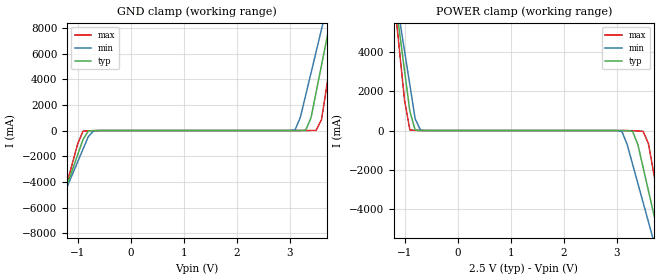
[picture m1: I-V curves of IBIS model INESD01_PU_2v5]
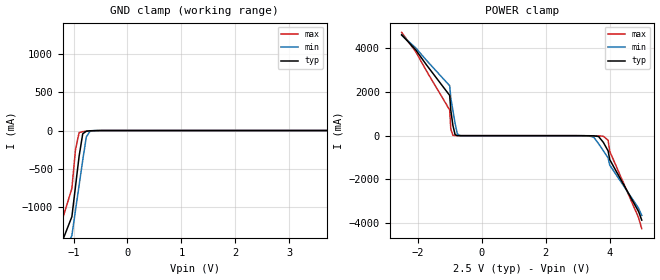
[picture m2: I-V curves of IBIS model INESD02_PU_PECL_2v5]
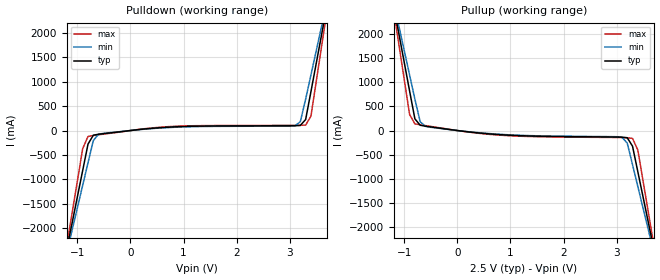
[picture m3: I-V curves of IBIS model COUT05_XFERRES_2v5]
|   This file is an IBIS representation of the   |
|   Integrated Devices Technology, Inc.   |
|   ICS83947I-147   |
|   Low Skew, 1-to-9 LVCMOS/LVTTL Fanout Buffer   |
[IBIS Ver]   4.1
[File name]   83947i_147.ibs
[File Rev]   1.0
[Date]   12 Jun 2009 | Last modified
|   July 26 2002 | Generated
[Source]   Originated at Integrated Devices Technology, Inc.
[Disclaimer]
IDT hereby grants the user of this IBIS model a non-exclusive,
nontransferable license to use this IBIS model under the following terms.
Before using this IBIS model, the user should read this license.
If the user does not accept these terms,  the IBIS model should be
returned to IDT within 30 days.
   The user is granted this license only to use the IBIS model and
is not granted rights to sell, load, rent, lease or license the IBIS
model in whole or in part, or in modified form to anyone other than
user. User may modify the IBIS model to suit its specific
applications but rights to derivative works and such modifications
shall belong to IDT.
   This IBIS model is provided on an "AS IS" basis and IDT makes
absolutely no warranty with respect to the information contained
herein. IDT DISCLAIMS AND CUSTOMER WAIVES ALL WARRANTIES, EXPRESS
OR IMPLIED, INCLUDING WARRANTIES OF MERCHANTABILITY OR FITNESS FOR
A PARTICULAR PURPOSE. The entire risk as to quality and performance
is with the Customer. ACCORDINGLY, IN NO EVENT SHALL THE COMPANY BE
LIABLE FOR ANY DAMAGES, WHETHER IN CONTRACT OR TORT,INCLUDING ANY
LOST PROFITS OR OTHER INCIDENTAL, CONSEQUENTIAL, EXEMPLARY, OR
PUNITIVE DAMAGES ARISING OUT OF THE USE OR APPLICATION OF THE IBIS
model provided in this package. Further, IDT reserves the right to
make changes without notice to any product herein to improve
reliability, function, or design. IDT does not convey any license
under patent rights or any other intellectual property rights,
including those of third parties.
   IDT is not obligated to provide maintenance or support
for the licensed IBIS model.
[Copyright]   Copyright 2002 by Integrated Devices Technology, Inc.
[Component]   ICS83947I-147
[Manufacturer] Integrated Devices Technology, Inc.
[Package]
|LQFP32
|lead + wire   typ   min   max
R_pkg   220.4m   212.5m   238m
L_pkg   1.841n   1.708n   1.974n
C_pkg   0.316p   0.2907p   0.33p
[Pin] signal_name   model_name   R_pin   L_pin   C_pin
1   GND   GND   238m   1.974n   0.330p
2   CLK_SEL   INESD01_PU   225m   1.841n   0.311p
3   CLK0   INESD02_PU_PECL 218m   1.7745n   0.301p
4   CLK1   INESD02_PU_PECL 213m   1.708n   0.291p
5   CLK_EN   INESD01_PU   213m   1.708n   0.291p
6   OE   INESD01_PU   218m   1.7745n   0.301p
7   VDD   POWER   225m   1.841n   0.311p
8   GND   GND   238m   1.974n   0.330p
9   GND   GND   238m   1.974n   0.330p
10   VDDO   POWER   225m   1.841n   0.311p
11   Q8   COUT05_XFERRES  218m   1.7745n   0.301p
12   GND   GND   213m   1.708n   0.291p
13   Q7   COUT05_XFERRES  213m   1.708n   0.291p
14   VDDO   POWER   218m   1.7745n   0.301p
15   Q6   COUT05_XFERRES  225m   1.841n   0.311p
16   GND   GND   238m   1.974n   0.330p
17   GND   GND   238m   1.974n   0.330p
18   VDDO   POWER   225m   1.841n   0.311p
19   Q5   COUT05_XFERRES  218m   1.7745n   0.301p
20   GND   GND   213m   1.708n   0.291p
21   Q4   COUT05_XFERRES  213m   1.708n   0.291p
22   VDDO   POWER   218m   1.7745n   0.301p
23   Q3   COUT05_XFERRES  225m   1.841n   0.311p
24   GND   GND   238m   1.974n   0.330p
25   GND   GND   238m   1.974n   0.330p
26   Q2   COUT05_XFERRES  225m   1.841n   0.311p
27   VDDO   POWER   218m   1.7745n   0.301p
28   Q1   COUT05_XFERRES  213m   1.708n   0.291p
29   GND   GND   213m   1.708n   0.291p
30   Q0   COUT05_XFERRES  218m   1.7745n   0.301p
31   VDDO   POWER   225m   1.841n   0.311p
32   GND   GND   238m   1.974n   0.330p
[Model Selector] INESD01_PU
INESD01_PU_2v5  Buffer selection for 2v5
INESD01_PU_3v3  Buffer selection for 3v3
[Model Selector] INESD02_PU_PECL
INESD02_PU_PECL_2v5  Buffer selection for 2v5
INESD02_PU_PECL_3v3  Buffer selection for 3v3
[Model Selector] COUT05_XFERRES
COUT05_XFERRES_2v5  Buffer selection for 2v5
COUT05_XFERRES_3v3  Buffer selection for 3v3
| Models and submodels in the file (6): INESD01_PU_2v5 (Input), INESD02_PU_PECL_2v5 (Input), COUT05_XFERRES_2v5 (Output), INESD01_PU_3v3 (Input), INESD02_PU_PECL_3v3 (Input), COUT05_XFERRES_3v3 (Output)
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[Model] INESD01_PU_2v5
Model_type   Input
Polarity   Non-Inverting
Vinl = 1.4V
Vinh = 1.85V
|   typ   min   max
C_comp   2pF   1.5pF   2.5pF
|   typ   min   max
[Voltage range]  2.5V   2.375V   2.625V
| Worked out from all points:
|   GND clamp passes 1 mA (typ) near -0.54 V on its own axis
|   POWER clamp passes 1 mA (typ) near -0.66 V on its own axis
[GND_clamp]
|Voltage   I(typ)   I(min)   I(max)
-2.5V     -19.6A     -17.18A    -23.67A
-1.6V     -8.969A    -8.332A    -10.1A
-1.5V     -7.788A    -7.349A    -8.588A
-900mV    -707.1mA   -1.46A     -57.43mA
-700mV    -7.027mA   -24.05mA   -13.28mA
3.1V      199.2uA    53.94mA    11.78uA
3.3V      28.4mA     2.748A     652.4uA
3.5V      3.045A     6.192A     15.72mA
3.6V      5.115A     7.914A     872.4mA
3.7V      7.185A     9.638A     3.52A
3.9V      11.33A     13.09A     8.818A
5V        34.14A     32.07A     37.99A
[POWER_clamp]
|Voltage   I(typ)   I(min)   I(max)
-1.5V     9.257A     9.207A     9.48A
-1.2V     7.185A     7.484A     6.83A
-1.1V     5.115A     5.761A     4.182A
-900mV    976.9mA    2.318A     34.23mA
-700mV    1.582mA    24.31mA    1.044mA
3.1V      -2.107mA   -51.03mA   -534.5uA
3.3V      -35.62mA   -1.705A    -10.86mA
3.5V      -1.886A    -3.666A    -39.41mA
3.6V      -3.066A    -4.647A    -666.9mA
3.8V      -5.426A    -6.612A    -3.684A
3.9V      -6.607A    -7.595A    -5.193A
5V        -19.6A     -18.41A    -21.79A
[Model] INESD02_PU_PECL_2v5
Model_type   Input
Polarity   Non-Inverting
Vinl = .8V
Vinh =  2V
|   typ   min   max
C_comp   2pF   1.5pF   2.5pF
|   typ   min   max
[Voltage range]  2.5V   2.375V   2.625V
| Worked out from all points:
|   GND clamp passes 1 mA (typ) near -0.59 V on its own axis
|   POWER clamp passes 1 mA (typ) near -0.70 V on its own axis
[GND_clamp]
|Voltage   I(typ)   I(min)   I(max)
-2.5V     -3.894A    -3.674A    -4.294A
-1.25V    -1.521A    -1.7A      -1.261A
-1.031V   -1.125A    -1.372A    -755.3mA
-896.9mV  -335.4mA   -714.7mA   -27.06mA
-695.9mV  -3.401mA   -10.7mA    -6.467mA
3.995V    711.6uA    10.32mA    481.3uA
4.062V    4.029mA    88.04mA    1.401mA
4.129V    40.44mA    547.3mA    3.341mA
4.196V    445.8mA    1.124A     14.79mA
4.263V    1.139A     1.7A       275.9mA
4.5V      1.832A     2.277A     1.163A
5V        3.219A     3.431A     2.937A
[POWER_clamp]
|Voltage   I(typ)   I(min)   I(max)
-2.5V     4.617A     4.594A     4.726A
-1V       1.842A     2.286A     1.176A
-963.9mV  1.149A     1.709A     289.6mA
-896.9mV  456.4mA    1.132A     15.33mA
-829.9mV  42.02mA    556.1mA    3.389mA
-762.9mV  4.159mA    91.01mA    1.421mA
-695.9mV  727.9uA    10.67mA    490.4uA
3.35V     -3.204mA   -9.193mA   -6.2mA
3.8V      -305mA     -689.5mA   -24.7mA
3.95V     -699.9mA   -1.018A    -211mA
4V        -1.095A    -1.346A    -716.4mA
5V        -3.863A    -3.649A    -4.255A
[Model] COUT05_XFERRES_2v5
Model_type   Output
Polarity   Non-Inverting
|   typ   min   max
C_comp   2pF   1.5pF   2.5pF
Vmeas = 1.25V
Rref = 50
Vref = 1.25V
|   typ   min   max
[Voltage range]   2.5V   2.375V   2.625V
[Pullup Reference]   2.5V   2.375V   2.625V
[Pulldown Reference]   0.0V   0.0V   0.0V
[GND Clamp Reference]   0.0V   0.0V   0.0V
[POWER Clamp Reference]   2.5V   2.375V   2.625V
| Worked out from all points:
|   slope of the pulldown table from 0 to 0.375 V, typ, clamps not added: 8.86 ohm
|   slope of the pullup table from 0 to 0.375 V, typ, clamps not added: 7.92 ohm
[pulldown]
|Voltage   I (typ)   I (min)   I (max)
-2.5V     -9.407A    -8.467A    -10.89A
-1.2V     -2.429A    -2.497A    -2.347A
-1.1V     -1.891A    -2.038A    -1.688A
-900mV    -815.3mA   -1.118A    -369.3mA
-800mV    -277.7mA   -658.8mA   -121mA
-600mV    -75.94mA   -74.93mA   -86.3mA
3.1V      97.86mA    96.58mA    105.9mA
3.3V      225.3mA    641.2mA    111.8mA
3.4V      794.9mA    1.136A     294.5mA
3.6V      1.955A     2.127A     1.718A
3.7V      2.536A     2.623A     2.431A
5V        10.13A     9.107A     11.75A
[pullup]
|Voltage   I (typ)   I (min)   I (max)
-2.5V     10.24A     9.216A     11.88A
-1.2V     2.591A     2.667A     2.502A
-1.1V     2.002A     2.164A     1.78A
-900mV    823.6mA    1.156A     334.8mA
-800mV    243.2mA    652.3mA    139.1mA
-600mV    90.17mA    86.22mA    102.1mA
3.1V      -138.3mA   -138.9mA   -146.3mA
3.3V      -324.7mA   -709.4mA   -163.3mA
3.4V      -856.2mA   -1.163A    -404.9mA
3.6V      -1.922A    -2.073A    -1.713A
3.7V      -2.455A    -2.529A    -2.368A
5V        -9.405A    -8.469A    -10.89A
[Ramp]
|   typ   min   max
dV/dt_r   1.50/0.6n   1.50/0.80n   1.50/0.4n
dV/dt_f   1.50/0.6n   1.50/0.80n   1.50/0.4n
